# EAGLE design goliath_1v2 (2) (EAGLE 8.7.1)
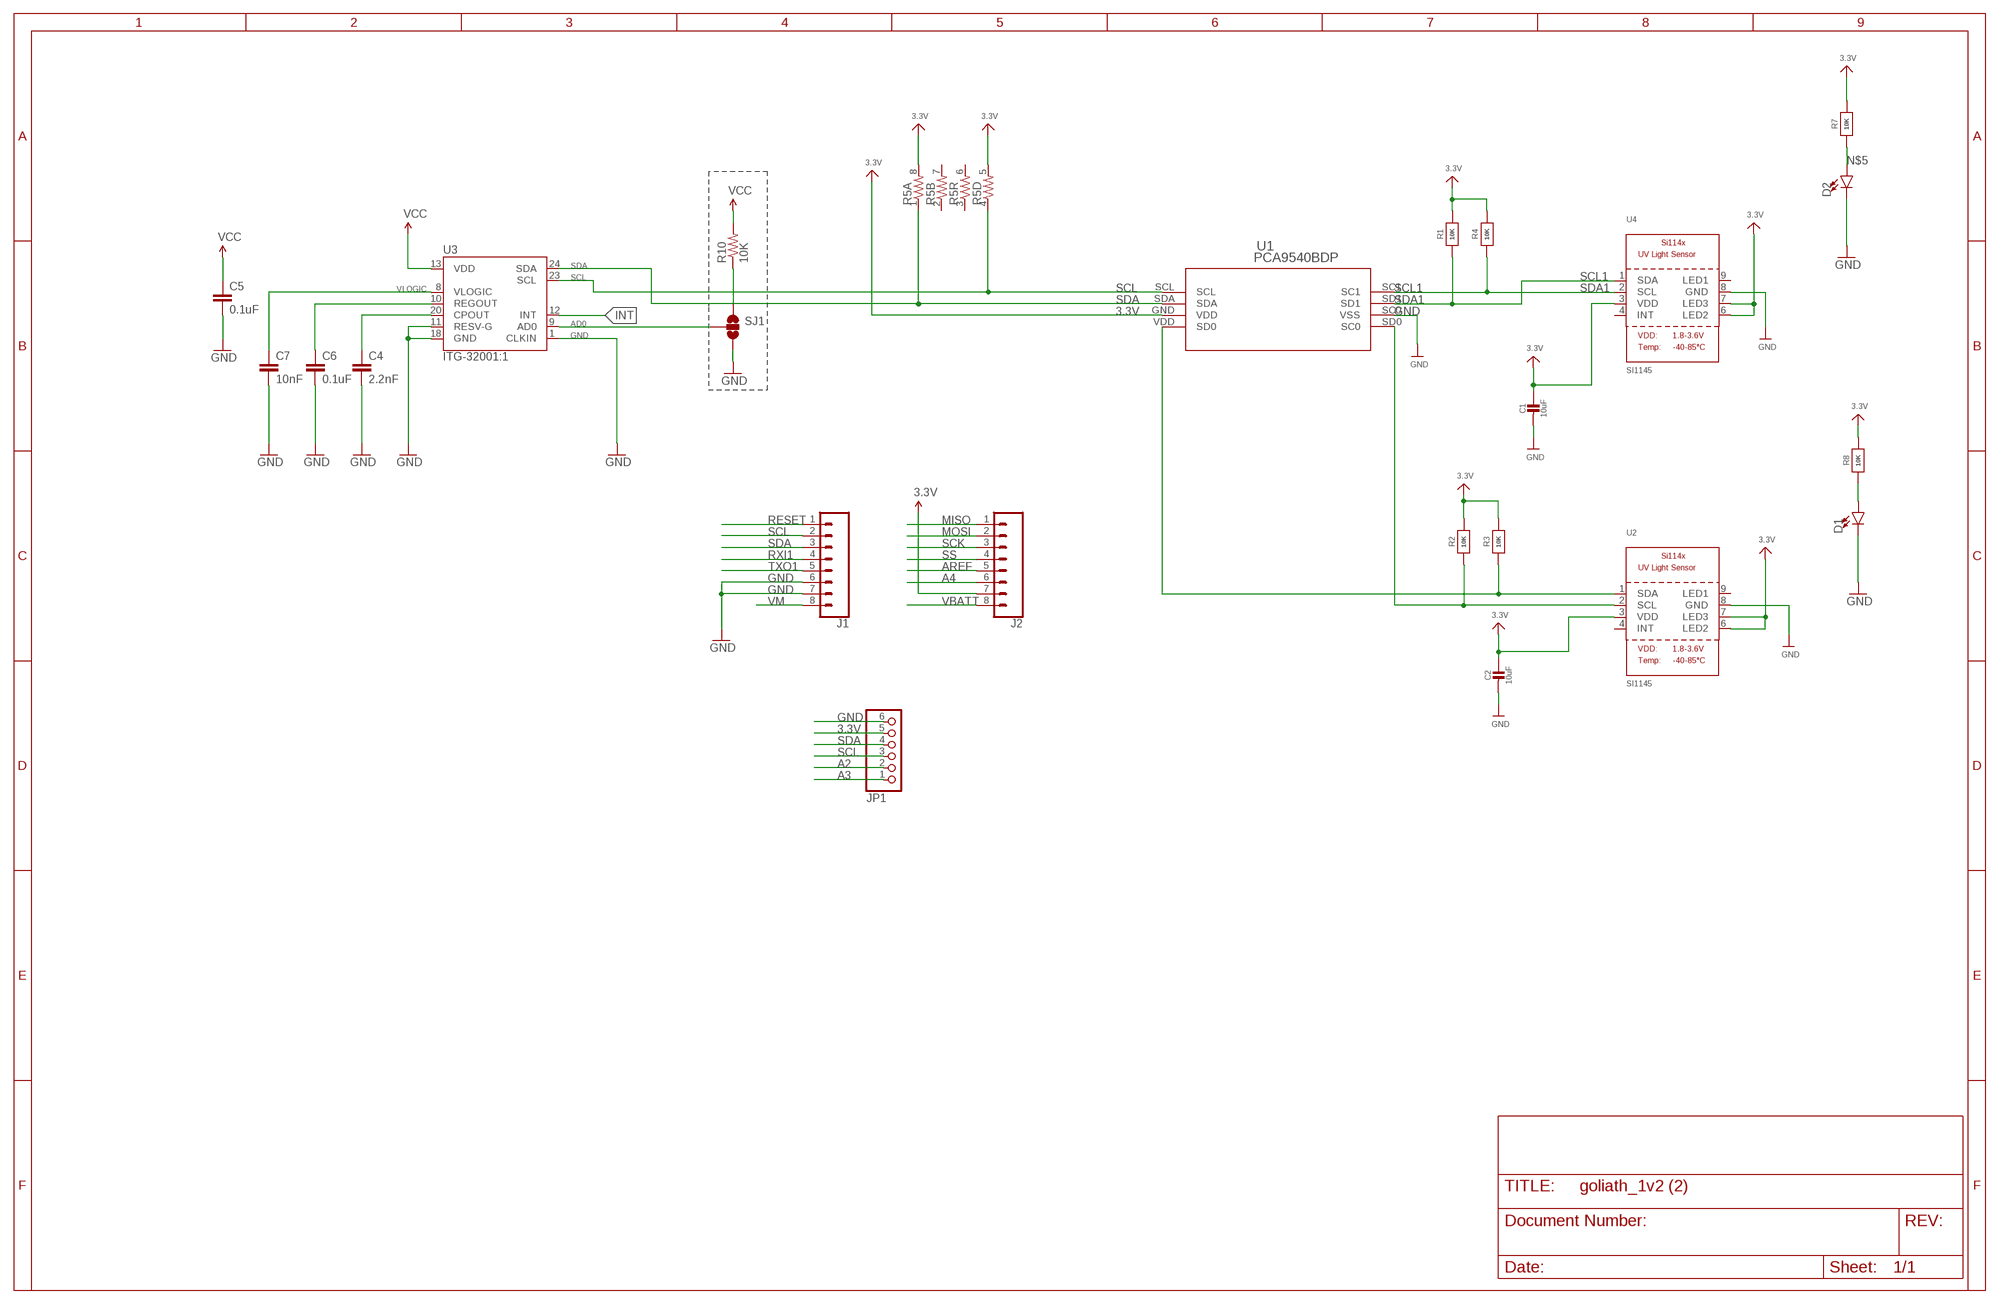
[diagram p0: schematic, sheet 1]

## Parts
C1  10uF  CAP_CERAMIC_0603  [_0603]
C2  10uF  CAP_CERAMIC_0603  [_0603]
C4  2.2nF  CAP0603-CAP  [0603-CAP]
C5  0.1uF  CAP0603-CAP  [0603-CAP]
C6  0.1uF  CAP0603-CAP  [0603-CAP]
C7  10nF  CAP0603-CAP  [0603-CAP]
D1  LED5MM  [LED_5MM]
D2  LED5MM  [LED_5MM]
J1  CONN_08"  [1X08]
J2  CONN_08"  [1X08]
JP1  PINHD-1X6  [1X06]
R1  10K  RESISTOR_0603  [_0603]
R2  10K  RESISTOR_0603  [_0603]
R3  10K  RESISTOR_0603  [_0603]
R4  10K  RESISTOR_0603  [_0603]
R5  RESISTOR-ARRAY0603-ARV  [0603-ARV]
R7  10K  RESISTOR_0603  [_0603]
R8  10K  RESISTOR_0603  [_0603]
R10  10K  10KOHM1/10W1%(0603)0603  [0603-RES]
SJ1  SOLDERJUMPER_2WAYPASTE1&2  [SJ_3_PASTE1&2]
U1  PCA9540BDP  [SOT505-1]
U2  SI1145  SI114X  [SI114X]
U3  ITG-32001:1  [QFN-24_ITG3200_1:1]
U4  SI1145  SI114X  [SI114X]

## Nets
3.3V: C1.1 C2.1 C5.1 J2.7 JP1.5 R1.2 R2.2 R3.2 R4.2 R5.5 R5.8 R7.2 R8.2 R10.2 U1.GND(VDD) U2.3(VDD) U2.6(LED2) U2.7(LED3) U3.13(VDD) U4.3(VDD) U4.6(LED2) U4.7(LED3) ; supply symbol labelled VCC
A2: JP1.2
A3: JP1.1
A4: J2.6
AD0: SJ1.2 U3.9(AD0)
AREF: J2.5
GND [vcc]: C1.2 C2.2 C4.2 C5.2 C6.2 C7.2 D1.K(C) D2.K(C) J1.6 J1.7 JP1.6 SJ1.3 U1.SC0(VSS) U2.8(GND) U3.1(CLKIN) U3.11(RESV-G) U3.18(GND) U4.8(GND)
INT: U3.12(INT)
MISO: J2.1
MOSI: J2.2
N$1: D1.A R8.1
N$5: D2.A R7.1
N$6: C6.1 U3.10(REGOUT)
N$7: C4.1 U3.20(CPOUT)
N$8: R10.1 SJ1.1
RESET: J1.1
RXI1: J1.4
SCK: J2.3
SCL: J1.2 JP1.3 R5.4 U1.SCL U3.23(SCL)
SCL0: R2.1 U1.SD0(SC0) U2.2(SCL)
SCL1: R4.1 U1.SC1 U4.2(SCL)
SDA: J1.3 JP1.4 R5.1 U1.SDA U3.24(SDA)
SDA0: R3.1 U1.VDD(SD0) U2.1(SDA)
SDA1: R1.1 U1.SD1 U4.1(SDA)
SS: J2.4
TXO1: J1.5
VBATT: J2.8
VLOGIC: C7.1 U3.8(VLOGIC)
VM: J1.8
Unconnected: R5.2 R5.3 R5.6 R5.7 U2.4(INT) U2.9(LED1) U4.4(INT) U4.9(LED1)

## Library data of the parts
C1 C2 = microbuilder:CAP_CERAMIC: Ceramic Capacitors
C4-C7 = SparkFun:CAP: Capacitor
D1 D2 = SparkFun-LED:LED: LED (Generic)
J1 J2 = SparkFun-Connectors-8pin:CONN_08: Multi connection point. Often used as Generic Header-pin footprint for 0.1 inch spaced/style header connections On any of the 0.1 inch spaced packages, you can populate with these: Break Away Headers - Straight (PRT-00116) Break Away Male Headers - Right Angle (PRT-00553) Female Headers (PRT-00115)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; PROD_ID: CONN-08438
JP1 = pinhead:PINHD-1X6: PIN HEADER
R1-R4 R7 R8 = microbuilder:RESISTOR: Resistors
R5 = SparkFun-Resistors:RESISTOR-ARRAY: Array Chip Resistor Source: RS Component / Phycomp
R10 = SparkFun-Resistors:10KOHM1/10W1%(0603): RES-00824; PROD_ID: RES-00824
SJ1 = SparkFun:SOLDERJUMPER_2WAY: Solder Jumper 2 way solder jumper
U1 = 2channel:PCA9540BDP; MANUFACTURER_PART_NUMBER: PCA9540BDP; VENDOR: NXP
U2 U4 = microbuilder:SI114X: Si1145/1146/1147 Proximity/UV/Ambient Light Sensor 1145 = 1 LED, 1146 = 2 LED, 1147 = 3 LED Proximity: 1-50cm LEDs: 5.6-360mA each
U3 = SparkFun-DigitalIC:ITG-3200: ITG-3200 3-axis gyro, digital output, qfn24 package

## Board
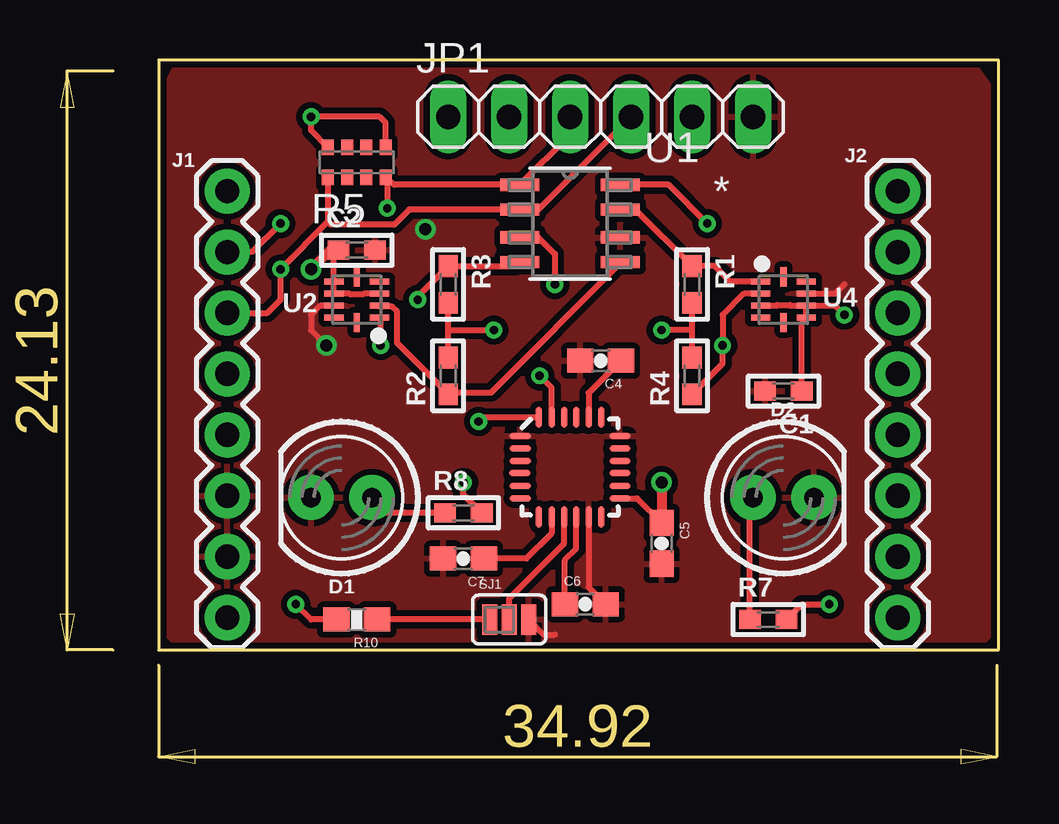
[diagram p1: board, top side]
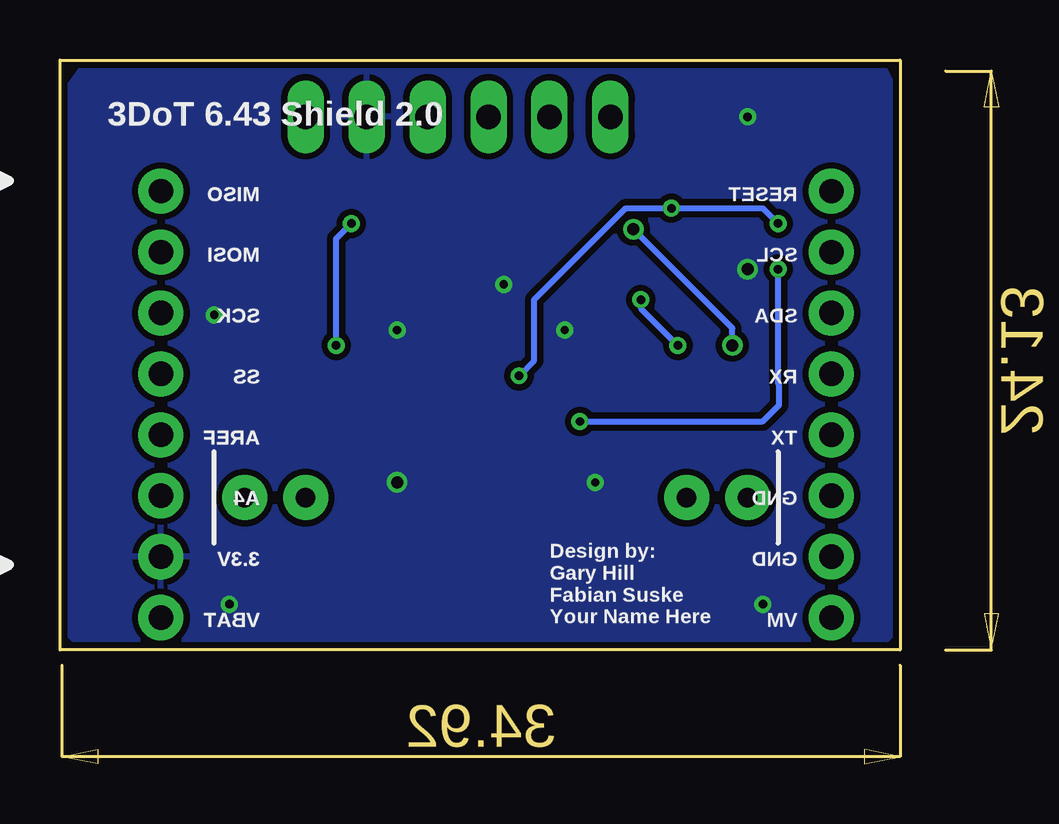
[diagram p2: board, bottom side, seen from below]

Size 39.11 x 29.34 mm. Coordinates in mm from the lower left corner, seen from the top.
Outline: 4.11,4.75 39.11,4.75 39.11,29.34 4.11,29.34 4.11,4.75
Copper layers (1*16): Top 0.035mm / dielectric 1.5mm / Bottom 0.035mm
Design rules "3DoT-2-layer-TIGHT": minimum track width 8mil, minimum drill 10mil, track to track 8mil, track to pad 8mil, pad to pad 8mil, via to via 8mil, smd to smd 8mil, copper to edge 10mil, drill to drill 8mil, minimum pad ring 10mil, minimum via ring 7mil, stop-mask expansion 4mil, vias tented up to drill 50mil, thermal gap 10mil

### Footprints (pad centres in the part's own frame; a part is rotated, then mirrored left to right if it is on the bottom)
_0603 = smd 0.9 x 0.8: 1 -0.762,0; 2 0.762,0
0603-CAP = smd 1.1 x 1: 1 -0.85,0; 2 0.85,0
LED_5MM = drill 0.813 pad 1.88: A -1.27,0; K 1.27,0
1X08 = drill 1.016 pad 1.88: 1 0,0; 2 2.54,0; 3 5.08,0; 4 7.62,0; 5 10.16,0; 6 12.7,0; 7 15.24,0; 8 17.78,0
1X06 = drill 1.016 long: 1 -6.35,0; 2 -3.81,0; 3 -1.27,0; 4 1.27,0; 5 3.81,0; 6 6.35,0
0603-ARV = smd 0.5 x 0.65: 1 -1.2,-0.625; 2 -0.4,-0.625; 3 0.4,-0.625; 4 1.2,-0.625; 5 1.2,0.625; 6 0.4,0.625; 7 -0.4,0.625; 8 -1.2,0.625
0603-RES = smd 1.1 x 1: 1 -0.85,0; 2 0.85,0
SJ_3_PASTE1&2 = smd 0.635 x 1.27: 1 -0.813,0; 2 0,0; 3 0.813,0
SOT505-1 = smd 1.626 x 0.508: GND -2.095,0.056; SC0 2.095,0.056; SC1 2.095,2.245; SCL -2.095,2.245; SD0 2.095,-0.975; SD1 2.095,1.214; SDA -2.095,1.214; VDD -2.095,-0.975
SI114X = smd 0.8 x 0.26: 1 -0.95,0.75; 2 -0.95,0.25; 3 -0.95,-0.25; 4 -0.95,-0.75; 6 0.95,-0.75; 7 0.95,-0.25; 8 0.95,0.25; 9 0.95,0.75 | smd 0.26 x 0.8: 5 0,-0.95; 10 0,0.95
QFN-24_ITG3200_1:1 = smd 0.889 x 0.279: 1 -2.076,1.301; 2 -2.076,0.775; 3 -2.076,0.25; 4 -2.102,-0.25; 5 -2.076,-0.775; 6 -2.076,-1.301; 13 2.076,-1.301; 14 2.076,-0.775; 15 2.076,-0.25; 16 2.076,0.25; 17 2.076,0.775; 18 2.076,1.301 | smd 0.279 x 0.889: 7 -1.301,-2.076; 8 -0.775,-2.076; 9 -0.25,-2.076; 10 0.25,-2.076; 11 0.775,-2.076; 12 1.301,-2.076; 19 1.301,2.076; 20 0.775,2.076; 21 0.25,2.076; 22 -0.25,2.076; 23 -0.775,2.076; 24 -1.301,2.076

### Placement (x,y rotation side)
C1  30.14,15.54 180 top
C2  12.37,21.41 0 top
C4  22.52,16.81 180 top
C5  25.06,9.19 270 top
C6  21.89,6.65 0 top
C7  16.81,8.55 180 top
D1  11.73,11.09 180 top
D2  30.14,11.09 0 top
J1  6.97,23.87 270 top
J2  34.91,23.87 270 top
JP1  22.52,26.97 0 top
R1  26.34,19.98 270 top
R2  16.18,16.18 90 top
R3  16.18,19.98 270 top
R4  26.34,16.18 90 top
R5  12.37,25.07 0 top
R7  29.51,6.02 0 top
R8  16.81,10.46 0 top
R10  12.37,6.02 180 top
SJ1  18.71,6.02 0 top
U1  21.25,21.89 0 top
U2  12.37,19.35 180 top
U3  21.25,12.37 0 top
U4  30.14,19.35 0 top

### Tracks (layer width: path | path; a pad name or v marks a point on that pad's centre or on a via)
3.3V  (via drill 0.35, 0.5)
  Top 0.254: U4.7 U4.6 30.91,18.41 C1.1 | R2.2 16.18,18.08 | 16.18,18.08 R3.2 | R4.2 26.34,18.08 | 26.34,18.08 R1.2 | U2.3 12.66,19.6 12.63,19.57 12.1,19.57 12.07,19.6 U2.7 U2.6 11.41,21.1 11.73,21.41 C2.1 | 26.34,18.08 v25.06,18.08 | R8.2 16.81,11.22 v16.81,11.73 | R5.8 10.46,26.39 v10.46,26.97 13.32,26.97 13.57,26.72 R5.5 | 16.18,18.08 v18.08,18.08 | U4.3 29.85,19.1 29.88,19.13 30.41,19.13 30.44,19.1 U4.7 | U4.7 32.3,19.1 v32.69,18.71 | R7.2 30.91,6.65 v32.05,6.65 | R10.2 10.46,6.02 v9.82,6.65 | U1.GND 19.93,21.95 20.62,21.26 v20.62,19.98 | U3.13 24.04,11.06 C5.1
  Top 0.406: v25.06,11.73 C5.1 | v10.46,20.62 11.25,21.41 C2.1
  pour Bottom (isolate 0.254, rank 6): 4.11,5.75 5.11,4.75 38.11,4.75 39.11,5.75 39.11,27.71 37.95,29.34 4.95,29.34 4.11,27.71
AD0
  Top 0.254: U3.9 21,9.18 18.71,6.89 SJ1.2
GND  (via drill 0.5)
  Top 0.254: U2.8 10.85,19.1 10.46,18.71 10.46,18.08 v11.1,17.45 | U4.8 32.3,19.6 32.69,19.98 | U3.11 22.03,7.36 C6.2 | SJ1.3 20.16,5.38 20.62,5.38
  Bottom 0.254: v11.1,17.45 11.1,18.16 v15.22,22.29
  pour Top (isolate 0.254, rank 6): 5.11,4.75 38.11,4.75 39.11,5.75 39.11,27.71 37.95,29.34 4.95,29.34 4.11,27.71 4.11,5.75
N$1
  Top 0.254: R8.1 13.64,10.46 D1.A
N$5
  Top 0.254: R7.1 28.75,10.97 D2.A
N$6
  Top 0.254: U3.10 21.5,8.96 21.04,8.5 C6.1
N$7
  Top 0.254: C4.1 22.03,15.46 U3.20
N$8
  Top 0.254: SJ1.1 R10.1
SCL  (via drill 0.35)
  Top 0.254: R5.4 13.64,24.37 | 13.64,24.37 v13.64,23.16 | v9.19,22.53 8,21.33 J1.2 | 13.7,24.43 13.66,24.4 | 13.66,24.4 13.64,24.37 | 13.66,24.4 13.93,24.14 U1.SCL 21.25,26.23 JP1.3 | U3.23 20.48,15.68 v19.98,16.18
  Bottom 0.254: v9.19,22.53 9.82,23.16 v13.64,23.16 15.54,23.16 19.35,19.35 19.35,16.81 v19.98,16.18
SCL0
  Top 0.254: R2.1 16.11,15.48 | 16.11,15.48 14.05,17.54 14.05,18.87 13.85,19.06 13.36,19.06 U2.2 | 16.11,15.48 17.96,15.48 23.35,20.86 U1.SD0
SCL1  (via drill 0.35)
  Top 0.254: 26.34,15.62 R4.1 27.61,16.68 v27.61,17.45 27.61,18.71 28.49,19.6 U4.2 | v26.97,22.53 25.36,24.14 U1.SC1
  Bottom 0.254: v27.61,17.45 27.61,21.89 v26.97,22.53
SDA  (via drill 0.35)
  Top 0.254: 11.16,22.6 v9.19,20.62 9.19,19.35 8.63,18.79 J1.3 | R5.1 11.16,22.6 | U3.24 17.62,14.44 v17.45,14.27 | JP1.4 19.93,23.1 U1.SDA 14.55,23.1 13.92,22.48 11.28,22.48 11.16,22.6
  Bottom 0.254: v17.45,14.27 9.82,14.27 9.14,14.95 9.14,15.82 9.19,15.87 v9.19,20.62
SDA0  (via drill 0.35)
  Top 0.254: v14.91,19.35 14.91,19.48 R3.1 18.99,20.75 U1.VDD | v13.36,17.45 13.36,18.55 U2.1
  Bottom 0.254: v14.91,19.35 14.91,18.99 v13.36,17.45
SDA1
  Top 0.254: U4.1 27.93,20.1 27.28,20.75 R1.1 23.98,23.1 U1.SD1
VLOGIC
  Top 0.254: U3.8 20.48,9.61 19.43,8.55 C7.1

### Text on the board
bPlace: 3DoT 6.43 Shield 2.0 | Design by: / Gary Hill / Fabian Suske / Your Name Here | RESET / / SCL / / SDA / / RX / / TX / / GND / / GND / / VM | MISO / / MOSI / / SCK / / SS / / AREF / / A4 / / 3.3V / / VBAT | MISO / / MOSI / / SCK / / SS / / AREF / / A4 / / 3.3V / / VBAT
Document: 3DoT Shield 1.0 / for 3DoT 6.12 / March 12, 2018 / / Designed by: / Fabian Suske fabiansuske@hotmail.de / / Deigned in: / Germany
